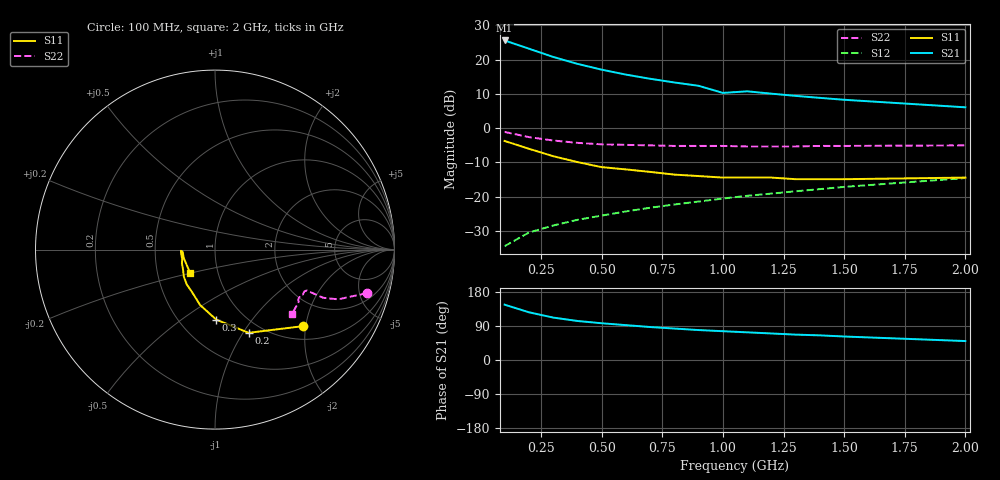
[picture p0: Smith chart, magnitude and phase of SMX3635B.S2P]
! HSMX-3635 Common Emitter
! Vce=10V Ic=10ma
# ghz s ma r 50
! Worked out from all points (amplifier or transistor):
!   16 points, 100 MHz to 2 GHz, reference 50 ohm
!   highest |S21| = 25.6 dB at 100 MHz (marker M1)
!   |S21| within 3 dB of that: start of sweep to 225.2 MHz
!   unconditionally stable (mu >= 1): 749.7 MHz to end of sweep
!   at 300 MHz: K = 0.70, MSG = 24.6 dB, |S12| = -28.4 dB
!   at 900 MHz: K = 1.03, MAG = 15.8 dB, |S12| = -21.4 dB
!   at 2 GHz: K = 1.02, MAG = 9.5 dB, |S12| = -14.6 dB
!   lowest NFmin = 1.30 dB at 500 MHz
!   S11 on the Smith chart (normalised r, x): 100 MHz: 1.31, -1.93; 200 MHz: 0.86, -1.06; 300 MHz: 0.74, -0.69; 2 GHz: 0.73, -0.20
0.1  0.65 -41.0  18.97 146.0  0.019 72.0  0.88 -16.0
0.2  0.5 -68.0  14.4 126.0  0.03 65.0  0.74 -22.0
0.3  0.39 -89.0  10.92 112.0  0.038 64.0  0.66 -24.0
0.4  0.32 -105.0  8.65 103.0  0.046 65.0  0.61 -24.0
0.5  0.27 -118.0  7.12 97.0  0.053 67.0  0.58 -24.0
0.6  0.25 -129.0  6.03 92.0  0.061 68.0  0.57 -24.0
0.7  0.23 -139.0  5.24 87.0  0.069 69.0  0.56 -24.0
0.8  0.21 -148.0  4.63 83.0  0.077 70.0  0.55 -25.0
0.9  0.2 -157.0  4.14 79.0  0.085 71.0  0.55 -26.0
1  0.19 -164.0  3.26 76.0  0.094 71.0  0.55 -27.0
1.1  0.19 -171.0  3.44 73.0  0.103 72.0  0.54 -28.0
1.2  0.19 -178.0  3.18 70.0  0.111 72.0  0.54 -30.0
1.3  0.18 -176.0  2.95 67.0  0.12 72.0  0.54 -31.0
1.4  0.18 -169.0  2.76 65.0  0.129 72.0  0.55 -32.0
1.5  0.18 -164.0  2.59 62.0  0.139 72.0  0.55 -33.0
2  0.19 -137.0  2.01 50.0  0.187 71.0  0.56 -40.0
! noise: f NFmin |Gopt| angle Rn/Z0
0.5  1.3  0.04  -29  1.06
1  1.4  0.18  -65  0.32
1.5  1.7  0.81  -14  0.06
2  2.3  0.57  -173  0.08
